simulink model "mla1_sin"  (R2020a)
settings: Solver=ode5  StartTime=0.0  StopTime=10  FixedStep=0.0001  RelTol=1e-4  EnableMultiTasking=on
PreLoadFcn:
  | MLA_Sensor1 = load('mla_sensor1.dat');
libraries: libmla x1

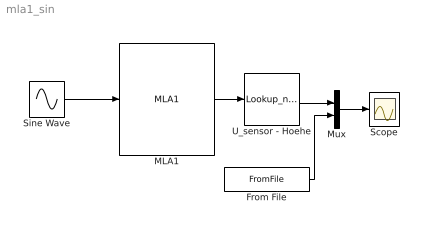
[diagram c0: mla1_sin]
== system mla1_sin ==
  From File : FromFile  FileName=mla_sin.mat  SampleTime=0
  MLA1 : libmla/MLA1  g=9.81  m=0.125  d_l=0.42  a=40691  b=0.0687  N=4.282
  Mux : Mux  Inputs=2
  Scope : Scope
  Sine Wave : Sin  Bias=2.5  Frequency=2  SampleTime=0
  U_sensor - Hoehe : Lookup_n-D  NumberOfTableDimensions=1  BreakpointsForDimension1=MLA_Sensor1(:,1)  Table=MLA_Sensor1(:,2)  RndMeth=Simplest
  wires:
  MLA1/1 -> U_sensor - Hoehe/1
  Sine Wave/1 -> MLA1/1
  U_sensor - Hoehe/1 -> Mux/1
  Mux/1 -> Scope/1
  From File/1 -> Mux/2
